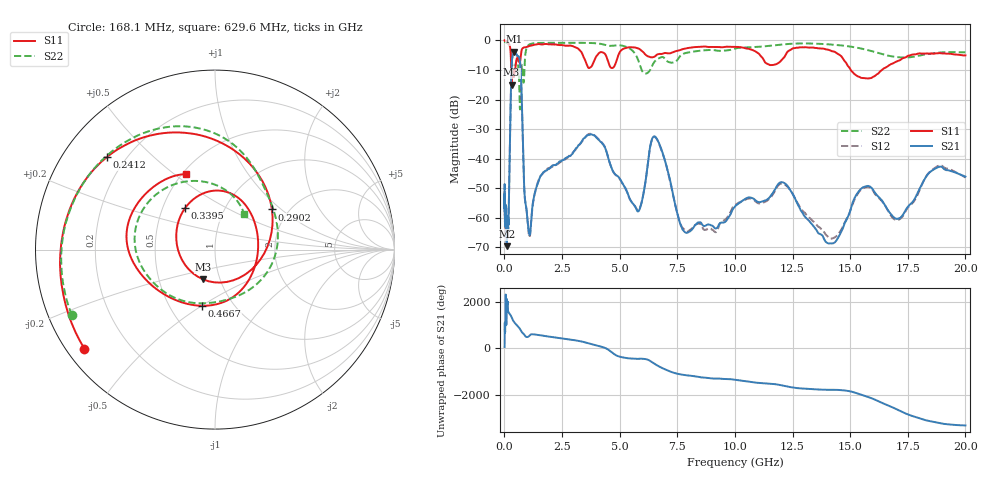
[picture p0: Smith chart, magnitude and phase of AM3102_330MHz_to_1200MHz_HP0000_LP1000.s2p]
! Date/Time: Tue, Sep 11, 2018 5:08 PM
! Network Analyzer: Agilent Technologies E8362B Rev: A.07.50.63
! Sweep from 0.010 to 20.000 GHz, 1601 Points, Sweep Type: LOG
! Power Supply: 4.950 V, 0.000 A
# Hz S DB R 50
!freq MagS11 AngS11 MagS21 AngS21 MagS12 AngS12 MagS22 AngS22
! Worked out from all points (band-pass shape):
!   1601 points, 10 MHz to 20 GHz, reference 50 ohm
!   highest |S21| = -3.81 dB at 432.6 MHz (marker M1); lowest = -69.7 dB at 103 MHz (marker M2)
!   |S21| within 3 dB of the highest: 326.7 MHz to 673.4 MHz (346.6 MHz wide, 69.3 % of centre)
!   lowest |S11| = -15.0 dB at 314.7 MHz (marker M3), VSWR 1.44, Z = 41.5 - j14.2 ohm
!   |S11| at or under -10 dB: 295.4 MHz to 348.2 MHz (52.77 MHz wide, 16.4 % of centre); 371.1 MHz to 463.9 MHz (92.79 MHz wide, 22.2 % of centre); 15.03 GHz to 16.38 GHz (1.351 GHz wide, 8.6 % of centre)
!   |S22| runs from -23.4 to -0.3 dB; largest |S21 - S12| = 0.012
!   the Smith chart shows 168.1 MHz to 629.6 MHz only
!   S11 on the Smith chart (normalised r, x): 168.1 MHz: 0.05, -0.34; 241.2 MHz: 0.13, +0.36; 290.2 MHz: 1.65, +0.87; 339.5 MHz: 0.65, +0.32; 466.7 MHz: 0.72, -0.50; 629.6 MHz: 0.52, +0.55
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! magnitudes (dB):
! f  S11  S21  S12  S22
! 10 MHz  0.0  -50.3  -53.5  -0.3
! 35.55 MHz  0.0  -62.3  -60.8  -0.5
! 103 MHz  -0.3  -69.7  -61.5  -0.8
! 126.4 MHz  -0.4  -63.8  -64.0  -0.9
! 168.1 MHz  -0.8  -61.4  -65.0  -1.1
! 241.2 MHz  -2.0  -34.6  -34.7  -1.9
! 290.2 MHz  -8.2  -14.2  -14.3  -3.8
! 314.7 MHz  -15.0  -8.2  -8.2  -6.2
! 339.5 MHz  -10.9  -5.9  -6.0  -8.2
! 432.6 MHz  -11.7  -3.8  -3.9  -10.1
! 447.2 MHz  -10.8  -3.9  -3.9  -9.4
! 466.7 MHz  -9.9  -4.0  -4.0  -8.7
! 629.6 MHz  -7.0  -5.5  -5.6  -11.8
! 1.067 GHz  -1.9  -65.0  -66.2  -1.4
! 1.59 GHz  -1.3  -45.7  -45.7  -0.8
! 3.793 GHz  -8.7  -31.8  -31.7  -0.8
! 5.652 GHz  -2.4  -56.0  -56.0  -4.3
! 6.549 GHz  -5.3  -32.6  -32.8  -6.9
! 7.92 GHz  -2.6  -65.2  -64.8  -4.1
! 12.03 GHz  -6.6  -48.0  -48.5  -1.4
! 14.14 GHz  -3.4  -68.8  -67.1  -1.3
! 20 GHz  -5.1  -46.1  -46.4  -4.0
